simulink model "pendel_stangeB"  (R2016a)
settings: Solver=ode45  StartTime=0.0  StopTime=10  MaxStep=0.01  RelTol=1e-3
InitFcn:
  | init_pendelStange
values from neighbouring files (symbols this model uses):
  b = zeros(N, 1)    [fourierrechteck.m]    (also in init_lorenzC.m = 28; init_pendelStange.m = 0.2)
  g = 9.81    [init_pendelStange.m]
  l = 1    [init_pendelStange.m]    (also in sfun_pendelstangeanim.m = block.DialogPrm(2).Data)
  lv = 0.3    [init_pendelStange.m]    (also in sfun_pendelstangeanim.m = block.DialogPrm(3).Data)
  m = 1.0    (= 1)    [init_pendelStange.m]
  om0 = 0    [init_pendelStange.m]
  phi0 = 0.4*pi    (= 1.25663706144)    [init_pendelStange.m]
  phiS = -pi/6    (= -0.523598775598)    [init_pendelStange.m]    (also in sfun_pendelstangeanim.m = block.DialogPrm(1).Data)
libraries: simulink x1

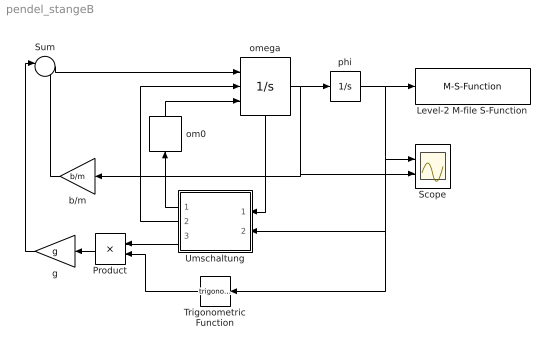
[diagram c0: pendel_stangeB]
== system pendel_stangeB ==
  note: .
  Level-2 M-file S-Function : M-S-Function  FunctionName=sfun_pendelstangeanim  Parameters=phiS, l, lv
  Product : Product  Inputs=/*
  Scope : Scope  NumInputPorts=2
  Sum : Sum  Inputs=|--
  Trigonometric Function : Trigonometry
  Umschaltung : Subsystem
  b/m : Gain  Gain=b/m
  g : Gain  Gain=g
  om0 : InitialCondition  Value=om0
  omega : Integrator  ExternalReset=either  InitialConditionSource=external  ShowStatePort=on
  phi : Integrator  InitialCondition=phi0
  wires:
  omega/1 -> phi/1, b/m/1, Scope/2
  phi/1 -> Trigonometric Function/1, Umschaltung/2(phi), Scope/1, Level-2 M-file S-Function/1
  Sum/1 -> omega/1
  b/m/1 -> Sum/2
  g/1 -> Sum/1
  Product/1 -> g/1
  Umschaltung/1(omega_neu) -> om0/1
  om0/1 -> omega/3
  omega/State -> Umschaltung/1(omega)
  Umschaltung/2(tr) -> omega/2
  Umschaltung/3(l) -> Product/1
  Trigonometric Function/1 -> Product/2

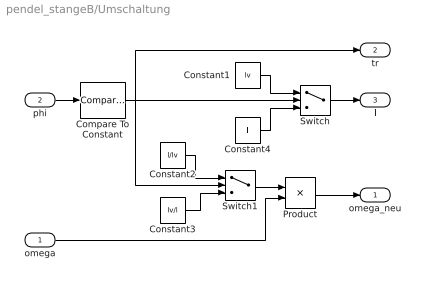
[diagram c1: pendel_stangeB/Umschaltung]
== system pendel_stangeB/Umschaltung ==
  omega : Inport
  phi : Inport  Port=2
  Compare To Constant : simulink/Logic and Bit Operations/Compare To Constant  SystemSampleTime=-1  relop=<=  const=phiS  LogicOutDataTypeMode=boolean
  Constant1 : Constant  Value=lv
  Constant2 : Constant  Value=l/lv
  Constant3 : Constant  Value=lv/l
  Constant4 : Constant  Value=l
  Product : Product
  Switch : Switch  Threshold=1
  Switch1 : Switch  Threshold=1
  omega_neu : Outport
  tr : Outport  Port=2
  l : Outport  Port=3
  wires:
  Compare To Constant/1 -> Switch/2, tr/1, Switch1/2
  Constant4/1 -> Switch/3
  Constant1/1 -> Switch/1
  phi/1 -> Compare To Constant/1
  Switch/1 -> l/1
  Constant2/1 -> Switch1/1
  Constant3/1 -> Switch1/3
  Switch1/1 -> Product/1
  Product/1 -> omega_neu/1
  omega/1 -> Product/2
